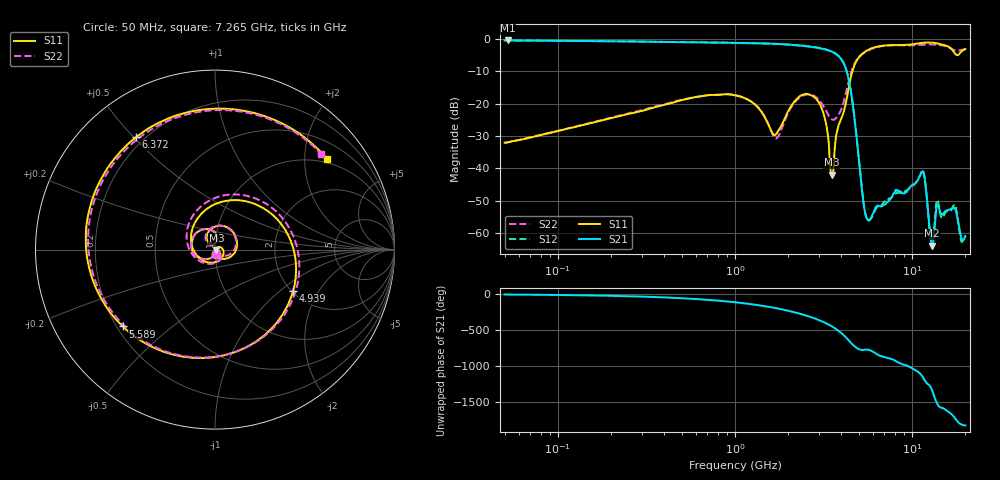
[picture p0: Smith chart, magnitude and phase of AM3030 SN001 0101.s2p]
# Hz S DB R 50
!freq MagS11 AngS11 MagS21 AngS21 MagS12 AngS12 MagS22 AngS22
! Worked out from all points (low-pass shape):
!   1601 points, 50 MHz to 20.05 GHz, reference 50 ohm
!   highest |S21| = -0.41 dB at 52.1 MHz (marker M1); lowest = -63.9 dB at 12.98 GHz (marker M2)
!   |S21| within 3 dB of the highest: start of sweep to 3.362 GHz
!   lowest |S11| = -41.9 dB at 3.525 GHz (marker M3), VSWR 1.02, Z = 50.7 - j0.32 ohm
!   |S11| at or under -10 dB: start of sweep to 4.607 GHz
!   |S22| runs from -32.2 to -1.6 dB; largest |S21 - S12| = 0.015
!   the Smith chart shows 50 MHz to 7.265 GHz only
!   S11 on the Smith chart (normalised r, x): 50 MHz: 1.01, -0.05; 4.939 GHz: 2.04, -1.24; 5.589 GHz: 0.22, -0.35; 6.372 GHz: 0.17, +0.51; 7.265 GHz: 0.90, +2.54
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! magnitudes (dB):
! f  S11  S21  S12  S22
! 50 MHz  -32.0  -0.4  -0.4  -32.2
! 52.1 MHz  -31.9  -0.4  -0.4  -32.0
! 135.9 MHz  -26.7  -0.6  -0.6  -26.6
! 369.6 MHz  -20.8  -0.8  -0.8  -20.6
! 1.005 GHz  -17.4  -1.2  -1.2  -17.3
! 1.704 GHz  -29.5  -1.4  -1.4  -30.7
! 2.182 GHz  -19.1  -1.8  -1.9  -19.5
! 2.722 GHz  -17.5  -2.4  -2.4  -17.3
! 3.198 GHz  -23.8  -3.1  -3.0  -21.2
! 3.525 GHz  -41.9  -3.9  -3.9  -24.8
! 4.3 GHz  -18.0  -10.3  -10.3  -15.3
! 4.939 GHz  -6.2  -33.6  -33.6  -6.0
! 5.589 GHz  -3.5  -55.7  -55.8  -3.7
! 6.372 GHz  -2.3  -51.6  -52.0  -2.5
! 7.265 GHz  -1.9  -50.4  -49.5  -2.0
! 7.402 GHz  -1.9  -49.9  -49.5  -1.9
! 11.47 GHz  -1.2  -41.0  -40.5  -1.8
! 12.98 GHz  -1.1  -63.9  -64.0  -1.6
! 13.99 GHz  -1.4  -51.2  -49.9  -1.8
! 17.39 GHz  -4.2  -52.2  -51.2  -3.5
! 18.95 GHz  -3.9  -61.2  -62.3  -3.4
! 20.05 GHz  -3.1  -60.9  -60.9  -3.2
